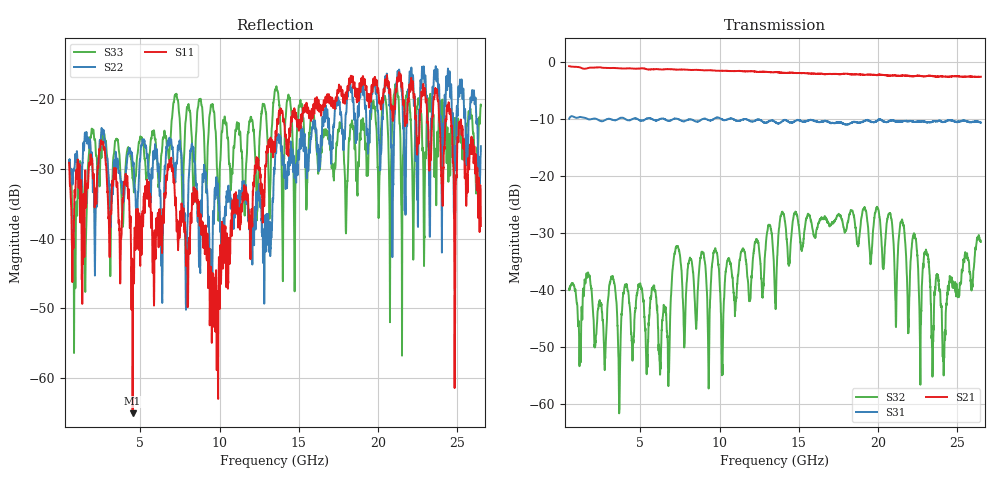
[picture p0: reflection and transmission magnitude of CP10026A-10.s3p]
#  HZ  S  DB  R  50.00
! Rohde & Schwarz Vector Network Analyzer
! Rohde-Schwarz,ZNB40-4Port,1311601084101679,3.45
! Created: UTC 2/9/2023, 11:29:52 AM
! freq[Hz]  db:S11  ang:S11  db:S12  ang:S12  db:S13  ang:S13
!  db:S21  ang:S21  db:S22  ang:S22  db:S23  ang:S23
!  db:S31  ang:S31  db:S32  ang:S32  db:S33  ang:S33
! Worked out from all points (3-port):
!   2601 points, 500 MHz to 26.5 GHz, reference 50 ohm
!   strongest paths, dB at 500 MHz, 7 GHz, 13.5 GHz, 20 GHz, 26.5 GHz:
!     S21: -0.7, -1.2, -1.7, -2.2, -2.6
!     S31: -9.9, -10.1, -10.5, -10.2, -10.6
!     S32: -39.9, -37.3, -41.4, -25.7, -31.6
!   lowest |S11| = -65.0 dB at 4.51 GHz (marker M1), VSWR 1.00, Z = 50.1 + j0.00741 ohm
!   |S11| at or under -10 dB: start of sweep to end of sweep
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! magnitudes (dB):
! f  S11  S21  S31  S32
! 500 MHz  -29.1  -0.7  -9.9  -39.9
! 4.51 GHz  -65.0  -1.1  -10.0  -52.2
! 6.85 GHz  -28.7  -1.2  -10.3  -48.1
! 7.27 GHz  -37.1  -1.3  -9.9  -32.6
! 9.79 GHz  -50.3  -1.5  -9.8  -33.3
! 10.17 GHz  -39.8  -1.5  -10.1  -54.6
! 13.5 GHz  -26.8  -1.7  -10.5  -41.4
! 19.94 GHz  -18.0  -2.3  -10.3  -25.4
! 24.16 GHz  -27.7  -2.5  -10.5  -53.7
! 26.5 GHz  -38.2  -2.6  -10.6  -31.6
